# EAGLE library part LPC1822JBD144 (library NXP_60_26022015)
32-bit ARM Cortex-M3 MCU; up to 1 MB flash and 136 kB SRAM; Ethernet, two High-speed USB, LCD, EMC The LPC185x/3x/2x/1x are ARM Cortex-M3 based microcontrollers for embedded applications. The ARM Cortex-M3 is a next generation core that offers system enhancements such as low power consumption, enhanced debug features, and a high level of support block integration. The LPC185x/3x/2x/1x operate at CPU frequencies of up to 180 MHz. The ARM Cortex-M3 CPU incorporates a 3-stage pipeline and uses a Harvard architecture with separate local instruction and data buses as well as a third bus for peripherals. The ARM Cortex-M3 CPU also includes an internal prefetch unit that supports speculative branching. The LPC185x/3x/2x/1x include up to 1 MB of flash and 136 kB of on-chip SRAM, 16 kB of EEPROM memory, a quad SPI Flash Interface (SPIFI), a State Configurable Timer (SCT) subsystem, two High-speed USB controllers, Ethernet, LCD, an external memory controller, and multiple digital and analog peripherals. AAL Eindhoven MK
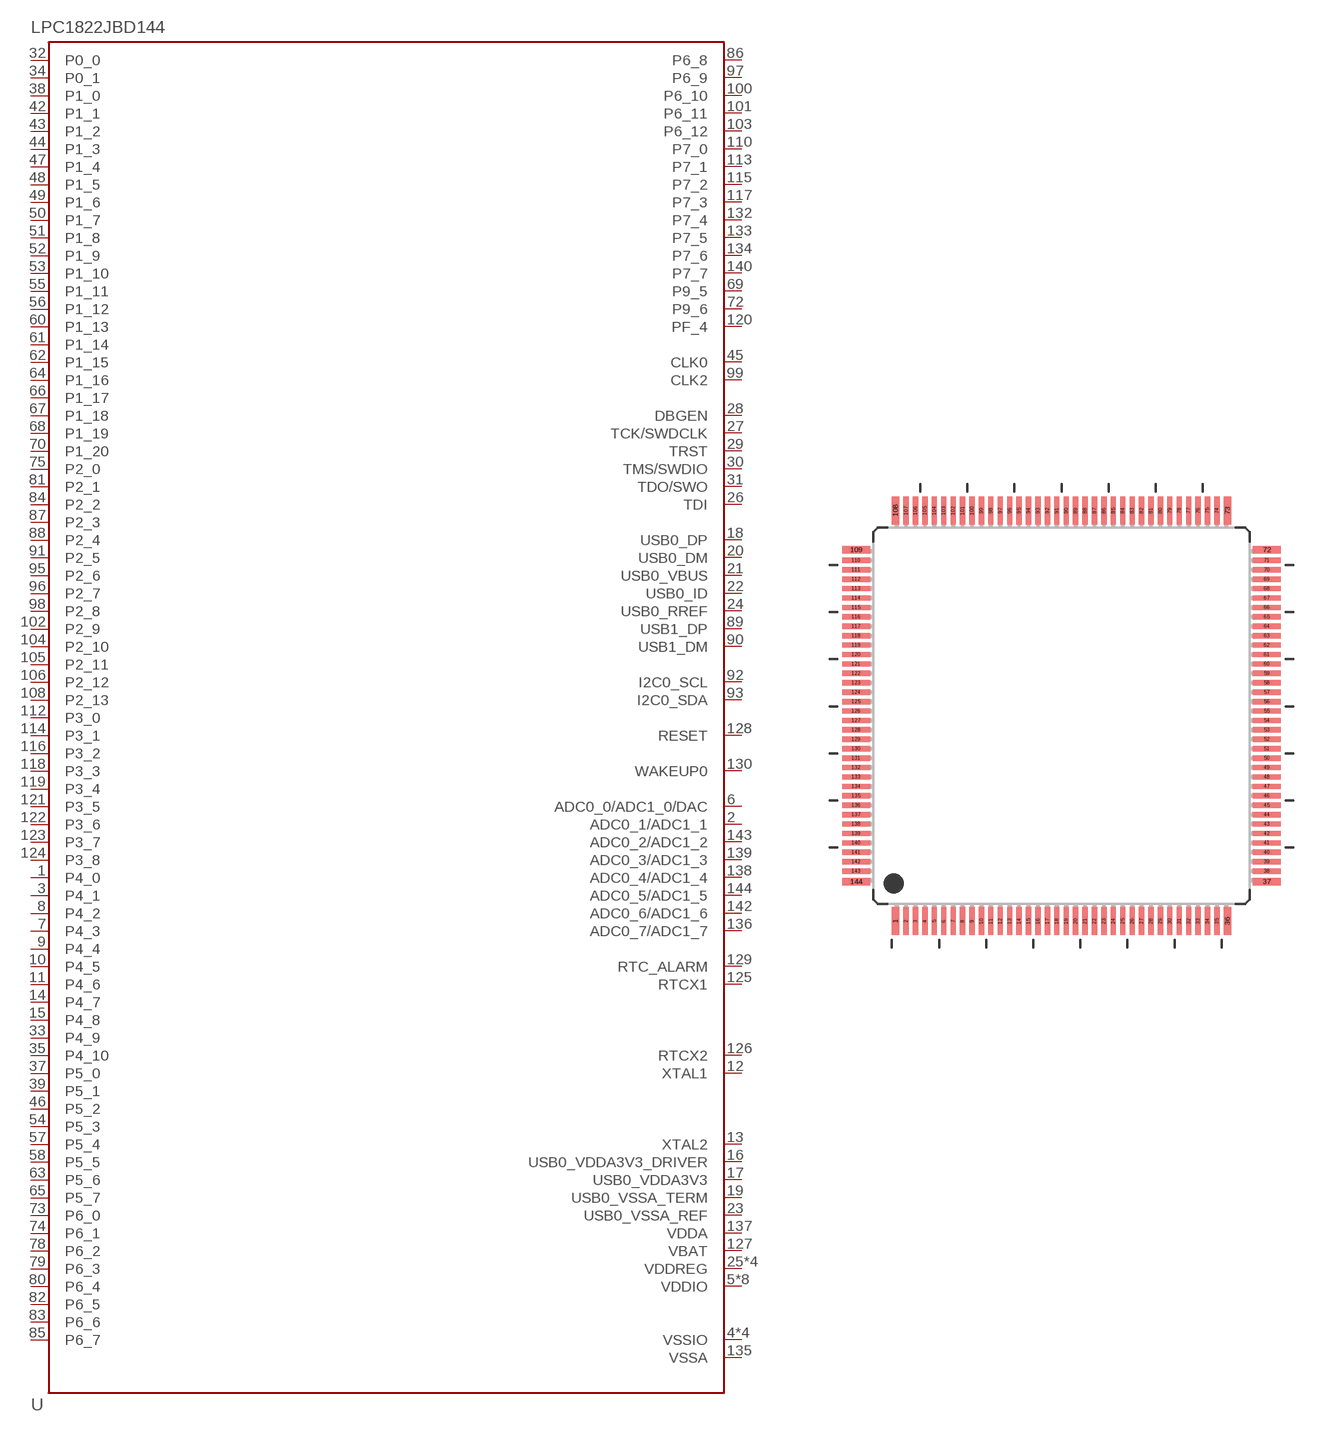
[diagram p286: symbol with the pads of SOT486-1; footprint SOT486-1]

Designator prefix U

## LPC1822JBD144 (ADC: 8; ETHERNET: no; FLASH: 512kB (1 bank); GPIO: 83; LCD: no; PWM: yes; QEI: no; SRAM: 104kB; TEMPERATURE_RANGE: -40 °C to +105 °C; USB0: Host/OTG; USB1: No)  [SOT486-1]
1  P4_0
2  ADC0_1/ADC1_1
3  P4_1
4  VSSIO
5  VDDIO
6  ADC0_0/ADC1_0/DAC
7  P4_3
8  P4_2
9  P4_4
10  P4_5
11  P4_6
12  XTAL1
13  XTAL2
14  P4_7
15  P4_8
16  USB0_VDDA3V3_DRIVER
17  USB0_VDDA3V3
18  USB0_DP
19  USB0_VSSA_TERM
20  USB0_DM
21  USB0_VBUS
22  USB0_ID
23  USB0_VSSA_REF
24  USB0_RREF
25  VDDREG
26  TDI
27  TCK/SWDCLK
28  DBGEN
29  TRST
30  TMS/SWDIO
31  TDO/SWO
32  P0_0
33  P4_9
34  P0_1
35  P4_10
36  VDDIO
37  P5_0
38  P1_0
39  P5_1
40  VSSIO
41  VDDIO
42  P1_1
43  P1_2
44  P1_3
45  CLK0
46  P5_2
47  P1_4
48  P1_5
49  P1_6
50  P1_7
51  P1_8
52  P1_9
53  P1_10
54  P5_3
55  P1_11
56  P1_12
57  P5_4
58  P5_5
59  VDDREG
60  P1_13
61  P1_14
62  P1_15
63  P5_6
64  P1_16
65  P5_7
66  P1_17
67  P1_18
68  P1_19
69  P9_5
70  P1_20
71  VDDIO
72  P9_6
73  P6_0
74  P6_1
75  P2_0
76  VSSIO
77  VDDIO
78  P6_2
79  P6_3
80  P6_4
81  P2_1
82  P6_5
83  P6_6
84  P2_2
85  P6_7
86  P6_8
87  P2_3
88  P2_4
89  USB1_DP
90  USB1_DM
91  P2_5
92  I2C0_SCL
93  I2C0_SDA
94  VDDREG
95  P2_6
96  P2_7
97  P6_9
98  P2_8
99  CLK2
100  P6_10
101  P6_11
102  P2_9
103  P6_12
104  P2_10
105  P2_11
106  P2_12
107  VDDIO
108  P2_13
109  VSSIO
110  P7_0
111  VDDIO
112  P3_0
113  P7_1
114  P3_1
115  P7_2
116  P3_2
117  P7_3
118  P3_3
119  P3_4
120  PF_4
121  P3_5
122  P3_6
123  P3_7
124  P3_8
125  RTCX1
126  RTCX2
127  VBAT
128  RESET
129  RTC_ALARM
130  WAKEUP0
131  VDDREG
132  P7_4
133  P7_5
134  P7_6
135  VSSA
136  ADC0_7/ADC1_7
137  VDDA
138  ADC0_4/ADC1_4
139  ADC0_3/ADC1_3
140  P7_7
141  VDDIO
142  ADC0_6/ADC1_6
143  ADC0_2/ADC1_2
144  ADC0_5/ADC1_5

## Footprint SOT486-1 (pad centres in mm)
SOT486-1 LQFP144: plastic low profile quad flat package; 144 leads; body 20 x 20 x 1.4 mm JEDEC: MS-026 IEC: 136E23
smd 0.4 x 1.5: 1 -8.81,-10.9; 36 8.81,-10.9; 73 8.81,10.9; 108 -8.81,10.9
smd 0.28 x 1.5: 2 -8.25,-10.9; 3 -7.75,-10.9; 4 -7.25,-10.9; 5 -6.75,-10.9; 6 -6.25,-10.9; 7 -5.75,-10.9; 8 -5.25,-10.9; 9 -4.75,-10.9; 10 -4.25,-10.9; 11 -3.75,-10.9; 12 -3.25,-10.9; 13 -2.75,-10.9; 14 -2.25,-10.9; 15 -1.75,-10.9; 16 -1.25,-10.9; 17 -0.75,-10.9; 18 -0.25,-10.9; 19 0.25,-10.9; 20 0.75,-10.9; 21 1.25,-10.9; 22 1.75,-10.9; 23 2.25,-10.9; 24 2.75,-10.9; 25 3.25,-10.9; 26 3.75,-10.9; 27 4.25,-10.9; 28 4.75,-10.9; 29 5.25,-10.9; 30 5.75,-10.9; 31 6.25,-10.9; 32 6.75,-10.9; 33 7.25,-10.9; 34 7.75,-10.9; 35 8.25,-10.9; 74 8.25,10.9; 75 7.75,10.9; 76 7.25,10.9; 77 6.75,10.9; 78 6.25,10.9; 79 5.75,10.9; 80 5.25,10.9; 81 4.75,10.9; 82 4.25,10.9; 83 3.75,10.9; 84 3.25,10.9; 85 2.75,10.9; 86 2.25,10.9; 87 1.75,10.9; 88 1.25,10.9; 89 0.75,10.9; 90 0.25,10.9; 91 -0.25,10.9; 92 -0.75,10.9; 93 -1.25,10.9; 94 -1.75,10.9; 95 -2.25,10.9; 96 -2.75,10.9; 97 -3.25,10.9; 98 -3.75,10.9; 99 -4.25,10.9; 100 -4.75,10.9; 101 -5.25,10.9; 102 -5.75,10.9; 103 -6.25,10.9; 104 -6.75,10.9; 105 -7.25,10.9; 106 -7.75,10.9; 107 -8.25,10.9
smd 1.5 x 0.4: 37 10.9,-8.81; 72 10.9,8.81; 109 -10.9,8.81; 144 -10.9,-8.81
smd 1.5 x 0.28: 38 10.9,-8.25; 39 10.9,-7.75; 40 10.9,-7.25; 41 10.9,-6.75; 42 10.9,-6.25; 43 10.9,-5.75; 44 10.9,-5.25; 45 10.9,-4.75; 46 10.9,-4.25; 47 10.9,-3.75; 48 10.9,-3.25; 49 10.9,-2.75; 50 10.9,-2.25; 51 10.9,-1.75; 52 10.9,-1.25; 53 10.9,-0.75; 54 10.9,-0.25; 55 10.9,0.25; 56 10.9,0.75; 57 10.9,1.25; 58 10.9,1.75; 59 10.9,2.25; 60 10.9,2.75; 61 10.9,3.25; 62 10.9,3.75; 63 10.9,4.25; 64 10.9,4.75; 65 10.9,5.25; 66 10.9,5.75; 67 10.9,6.25; 68 10.9,6.75; 69 10.9,7.25; 70 10.9,7.75; 71 10.9,8.25; 110 -10.9,8.25; 111 -10.9,7.75; 112 -10.9,7.25; 113 -10.9,6.75; 114 -10.9,6.25; 115 -10.9,5.75; 116 -10.9,5.25; 117 -10.9,4.75; 118 -10.9,4.25; 119 -10.9,3.75; 120 -10.9,3.25; 121 -10.9,2.75; 122 -10.9,2.25; 123 -10.9,1.75; 124 -10.9,1.25; 125 -10.9,0.75; 126 -10.9,0.25; 127 -10.9,-0.25; 128 -10.9,-0.75; 129 -10.9,-1.25; 130 -10.9,-1.75; 131 -10.9,-2.25; 132 -10.9,-2.75; 133 -10.9,-3.25; 134 -10.9,-3.75; 135 -10.9,-4.25; 136 -10.9,-4.75; 137 -10.9,-5.25; 138 -10.9,-5.75; 139 -10.9,-6.25; 140 -10.9,-6.75; 141 -10.9,-7.25; 142 -10.9,-7.75; 143 -10.9,-8.25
